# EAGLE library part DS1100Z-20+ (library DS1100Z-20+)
DS1100Z-20+, Delay Line, 5-Taps 500ns, 8-Pin SOIC Source: Datasheet
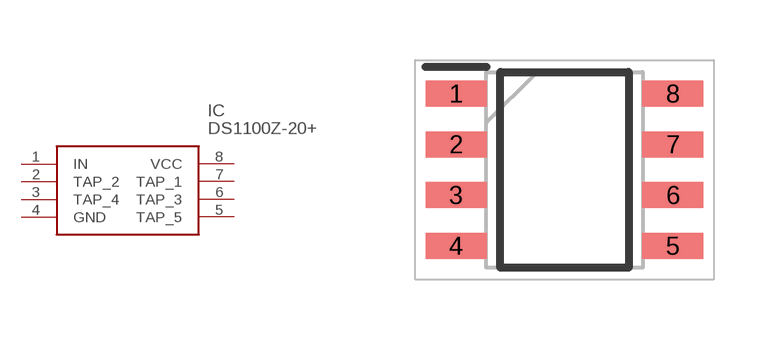
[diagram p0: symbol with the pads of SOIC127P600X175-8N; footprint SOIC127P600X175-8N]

Designator prefix IC

## DS1100Z-20+ (Description: DS1100Z-20+, Delay Line, 5-Taps 500ns, 8-Pin SOIC; Height: 1.75mm; Manufacturer_Name: Analog Devices; Manufacturer_Part_Number: DS1100Z-20+; Mouser_Part_Number: 700-DS1100Z-20; Mouser_Price-Stock: https://www.mouser.co.uk/ProductDetail/Analog-Devices-Maxim-Integrated/DS1100Z-20%2b?qs=0Y9aZN%252BMVCX5CJKJjF7c1Q%3D%3D)  [SOIC127P600X175-8N]
1  IN
2  TAP_2
3  TAP_4
4  GND
5  TAP_5
6  TAP_3
7  TAP_1
8  VCC

## Footprint SOIC127P600X175-8N (pad centres in mm)
S8+4
smd 1.525 x 0.65: 1 -2.712,1.905; 2 -2.712,0.635; 3 -2.712,-0.635; 4 -2.712,-1.905; 5 2.712,-1.905; 6 2.712,-0.635; 7 2.712,0.635; 8 2.712,1.905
